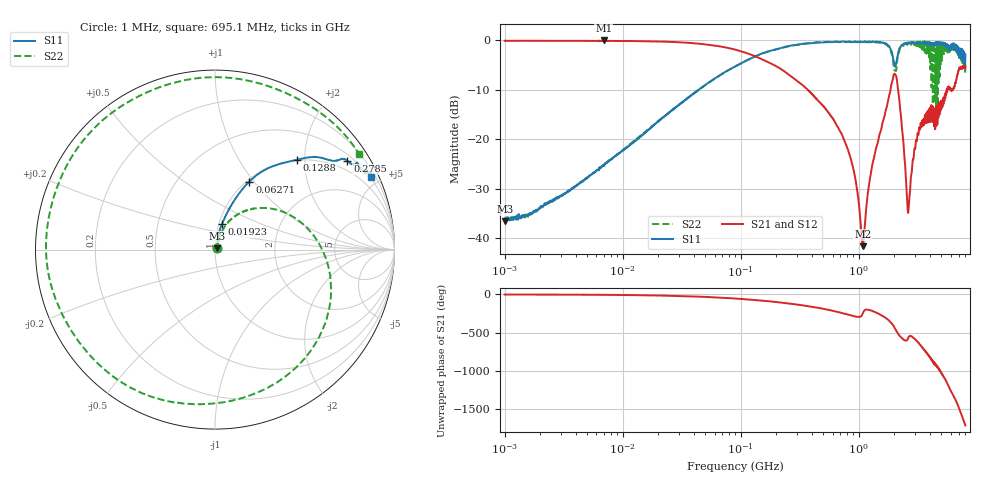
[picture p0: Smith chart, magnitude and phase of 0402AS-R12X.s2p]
!s-Parameter Generated by FASTRON Sdn. Bhd.
!FASTRON P/N : 0402AS-R12X
!Keysight Technologies: E5071C_MY46733604_B.14.02
!Date: Mon Dec 01 10:48:53 2025
!Version  :Rev00  Mon Dec 01 10:48:53 2025
!Data & Calibration Information:
!Freq  S11:SOLT2(ON)  S21:SOLT2(ON)  S12:SOLT2(ON)  S22:SOLT2(ON)
!PortZ  Port1:50+j0  Port2:50+j0
!When reading reference impedance value at option line is always used.
! Remarks : This data is being provided solely for informational purposes.
# Hz S dB R 50
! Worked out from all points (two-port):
!   1601 points, 1 MHz to 8 GHz, reference 50 ohm
!   highest |S21| = -0.05 dB at 6.912 MHz (marker M1); lowest = -41.6 dB at 1.081 GHz (marker M2)
!   |S21| within 3 dB of the highest: start of sweep to 126.3 MHz
!   lowest |S11| = -36.6 dB at 1.013 MHz (marker M3), VSWR 1.03, Z = 51.3 + j0.79 ohm
!   |S11| at or under -10 dB: start of sweep to 43.95 MHz
!   |S22| runs from -36.5 to -0.2 dB; largest |S21 - S12| = 0.015
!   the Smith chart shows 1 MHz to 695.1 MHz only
!   S11 on the Smith chart (normalised r, x): 1 MHz: 1.03, +0.02; 19.23 MHz: 1.04, +0.30; 62.71 MHz: 1.03, +0.95; 128.8 MHz: 0.99, +1.83; 278.5 MHz: 0.68, +3.16; 695.1 MHz: 0.46, +4.45
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1000000  -36.20 31.9  -0.12 -0.7  -0.12 -0.8  -36.40 31.8
1013202  -36.60 31.4  -0.12 -0.7  -0.12 -0.8  -36.30 30.9
4479405  -28.60 67.3  -0.13 -3.0  -0.12 -3.1  -28.60 66.4
6911657  -25.40 70.6  -0.05 -5.0  -0.15 -4.4  -25.30 67.3
1.923391e7  -16.70 74.6  -0.25 -12.8  -0.25 -12.7  -16.70 66.5
2.00676e7  -16.40 74.3  -0.26 -13.4  -0.26 -13.3  -16.30 65.9
6.270681e7  -7.45 63.2  -1.15 -38.9  -1.15 -38.8  -7.51 31.0
8.994653e7  -5.27 56.6  -1.90 -53.2  -1.89 -53.2  -5.28 10.0
1.287954e8  -3.40 47.7  -3.12 -71.5  -3.11 -71.5  -3.41 -16.9
2.784714e8  -1.03 33.8  -7.63 -126.0  -7.62 -126.0  -1.03 -110.0
4.006501e8  -0.60 27.7  -10.80 -162.0  -10.80 -162.0  -0.54 -176.0
6.950598e8  -0.38 25.1  -18.40 123.0  -18.40 123.0  -0.32 33.4
1.080879e9  -0.41 30.5  -41.60 112.0  -41.70 112.0  -0.35 -159.0
1.295411e9  -0.33 37.1  -25.40 145.0  -25.40 145.0  -0.42 95.6
1.48876e9  -0.40 41.8  -19.30 104.0  -19.30 103.0  -0.49 2.9
1.7949e9  -1.11 44.7  -11.50 19.6  -11.50 19.5  -1.43 -154.0
2.281485e9  -1.14 80.2  -15.30 156.0  -15.30 156.0  -1.56 -4.0
2.648292e9  -0.67 83.4  -33.60 164.0  -33.60 164.0  -0.64 178.0
2.985754e9  -0.46 91.1  -21.90 132.0  -21.90 131.0  -0.71 1.6
3.345355e9  -0.54 99.1  -16.70 47.7  -16.70 47.4  -1.52 -177.0
3.710194e9  -0.75 107.0  -15.70 -30.9  -15.70 -31.4  -0.34 19.1
8e9  -2.86 -115.0  -5.48 77.2  -5.51 76.7  -4.95 115.0
